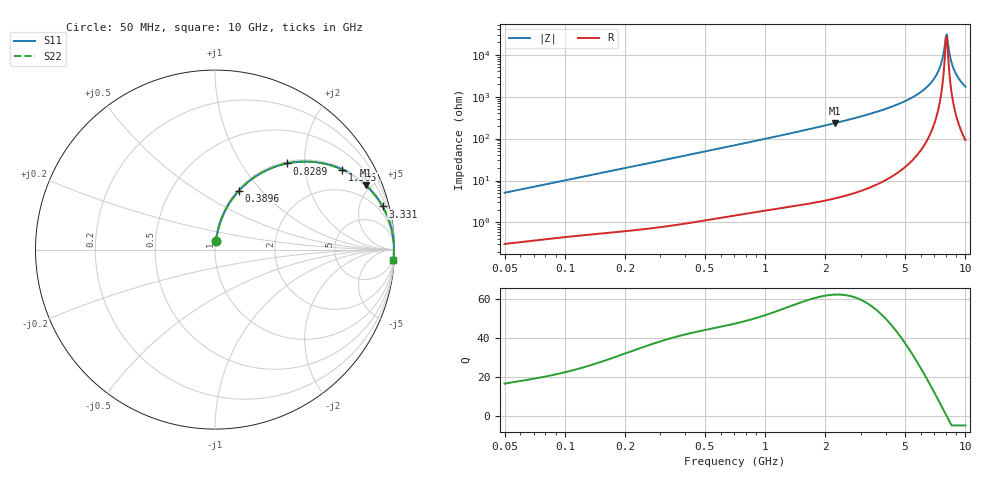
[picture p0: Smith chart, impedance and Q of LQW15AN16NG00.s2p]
!Murata Part Number: LQW15AN16NG00
!These Parameters are Measured in Series Mode Connection
!  o--[Z]--o
!Port1  Port2
!  o-------o
!Freq. Start=50[MHz] Stop=10[GHz], 401[Steps]
# Hz S RI R 50
!Freq.(Hz)	S 11(Real)	S 11(Imag)	S 21(Real)	S 21(Imag)	S 12(Real)	S 12(Imag)	S 22(Real)	S 22(Imag)
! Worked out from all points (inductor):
!   401 points, 50 MHz to 10 GHz, reference 50 ohm
!   read as one part in series: L = 16.1 nH near 51.34 MHz
!   highest Q = 62.3 at 2.239 GHz (marker M1), where L = 16.6 nH
!   self-resonance near 7.984 GHz
!   S11 on the Smith chart (normalised r, x): 50 MHz: 1.01, +0.10; 389.6 MHz: 1.02, +0.77; 828.9 MHz: 1.03, +1.63; 1.565 GHz: 1.05, +3.15; 3.331 GHz: 1.14, +7.73; 10 GHz: 3, -35
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5e7  0.00563 0.0505  0.9944 -0.0505  0.9944 -0.0505  0.00563 0.0505
1.214486e8  0.0191 0.1182  0.9809 -0.1182  0.9809 -0.1182  0.0191 0.1182
2.949953e8  0.084 0.2645  0.916 -0.2645  0.916 -0.2645  0.084 0.2645
3.896002e8  0.1342 0.329  0.8658 -0.329  0.8658 -0.329  0.1342 0.329
7.071068e8  0.3291 0.4595  0.6709 -0.4595  0.6709 -0.4595  0.3291 0.4595
8.289263e8  0.4014 0.4801  0.5986 -0.4801  0.5986 -0.4801  0.4014 0.4801
1.565451e9  0.709 0.4458  0.291 -0.4458  0.291 -0.4458  0.709 0.4458
1.717543e9  0.7478 0.426  0.2522 -0.426  0.2522 -0.426  0.7478 0.426
2.23851e9  0.8416 0.3572  0.1584 -0.3572  0.1584 -0.3572  0.8416 0.3572
3.330706e9  0.9336 0.2403  0.0664 -0.2403  0.0664 -0.2403  0.9336 0.2403
4.171863e9  0.9644 0.1752  0.0356 -0.1752  0.0356 -0.1752  0.9644 0.1752
5.583245e9  0.9875 0.0954  0.0125 -0.0954  0.0125 -0.0954  0.9875 0.0954
6.720828e9  0.9947 0.0467  0.00526 -0.0467  0.00526 -0.0467  0.9947 0.0467
7.37379e9  0.9965 0.0227  0.00353 -0.0227  0.00353 -0.0227  0.9965 0.0227
7.571744e9  0.9967 0.0158  0.00326 -0.0158  0.00326 -0.0158  0.9967 0.0158
7.878683e9  0.997 0.0055  0.00303 -0.0055  0.00303 -0.0055  0.997 0.0055
7.983737e9  0.997 0.00207  0.003 -0.00207  0.003 -0.00207  0.997 0.00207
8.198065e9  0.997 -0.0048  0.00301 0.0048  0.00301 0.0048  0.997 -0.0048
8.530394e9  0.9968 -0.0151  0.00322 0.0151  0.00322 0.0151  0.9968 -0.0151
8.876195e9  0.9964 -0.0255  0.00364 0.0255  0.00364 0.0255  0.9964 -0.0255
9.359165e9  0.9954 -0.0394  0.00457 0.0394  0.00457 0.0394  0.9954 -0.0394
1e10  0.9937 -0.057  0.00631 0.057  0.00631 0.057  0.9937 -0.057
